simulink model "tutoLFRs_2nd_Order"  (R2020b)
settings: Solver=VariableStepAuto  StartTime=0.0  StopTime=10.0  RelTol=1e-3
undefined symbols (not defined in the file): w, xi
libraries: RCTblocks x2

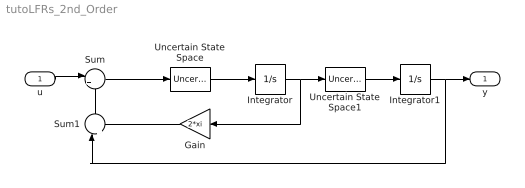
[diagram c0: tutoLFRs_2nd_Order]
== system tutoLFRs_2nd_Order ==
  u : Inport
  Gain : Gain  Gain=2*xi
  Integrator : Integrator
  Integrator1 : Integrator
  Sum : Sum  Inputs=|+-
  Sum1 : Sum  Inputs=|++
  Uncertain State Space : RCTblocks/Uncertain State Space  Tag=USS  USystem=ss(w)  UValue=[]  X0=[]  uX0=[]
  Uncertain State Space1 : RCTblocks/Uncertain State Space  Tag=USS  USystem=ss(w)  UValue=[]  X0=[]  uX0=[]
  y : Outport
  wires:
  Uncertain State Space/1 -> Integrator/1
  Integrator/1 -> Gain/1, Uncertain State Space1/1
  Uncertain State Space1/1 -> Integrator1/1
  Integrator1/1 -> Sum1/1, y/1
  u/1 -> Sum/1
  Sum/1 -> Uncertain State Space/1
  Sum1/1 -> Sum/2
  Gain/1 -> Sum1/2
